PROGRAM MAIN_SLOW
VAR
	iAxis                : USINT;	(* Axis index *)
	configurationManager : ConfigurationManager; (* The axis configuration FB *) 
	twincatEventTrialink : TL_TwinCatError;  (* Axis independent events of the library *)
	
END_VAR

(* ------------------------------------------- *)
(* Triamec Motion AG, 6340 Baar, Switzerland   *)
(* Sample Code may be adapted to customer need *)
(* ------------------------------------------- *)

configurationManager();
gTrialink.CallSlow();

gCommunicationReady	:= NOT gTrialink.error;
FOR iAxis:=1 TO N_AXES DO

	gAxes[iAxis].iAxis	:= iAxis;	(* logical axis number used in MAIN_FAST *)
	gAxes[iAxis].reset	:= gReset;	(* reset drive errors *)
	gAxes[iAxis].enable	:= gEnable;	(* set enable/disable *)
	gAxes[iAxis].couple	:= TRUE;	(* couple drive to CNC-pathplanner *)
	gAxes[iAxis].CallSlow(Trialink := gTrialink);
	
	gCommunicationReady	:= gCommunicationReady 	AND gAxes[iAxis].ready;

	gNciAxes[iAxis].Enable			  := gAxes[iAxis].enabled;
	gNciAxes[iAxis].followMe		  := gAxes[iAxis].followMe;
	gNciAxes[iAxis].Reset			  := (gReset AND gAxes[iAxis].error);
	gNciAxes[iAxis].TorquePermission  := gAxes[iAxis].coupled;
	gNciAxes[iAxis].CallSlow(axis := gAxes[iAxis].MC_axis);

END_FOR

END_PROGRAM
